FUNCTION_BLOCK MIS_Ctrl
VAR_INPUT
	wNode : WORD; //CANopen nodeID for motor
	ADSNetID : STRING(23); //ADS adress of CANopen master module
	lrUnitConversion : LREAL := 1.0; //Default conversion is 1
END_VAR
VAR_OUTPUT
	stMisMotori : stMisMotor; //Instance of the Mis motor structure
END_VAR
VAR
	bLastEnableMotor : BOOL;//Used to trigger motor enable state 
	iState: INT; //Current state of test
END_VAR

StateHandler(); //handle CANeopen FSA state 
stMisMotori.lrActualUnitPos := ANY_TO_LREAL(stMisMotori.diActualpos) / stMisMotori.lrUnitConversion;//Convert motorcount to units  


CASE iState OF
0:
	stMisMotori.wNodeId := wNode;
	stMisMotori.ADSNetID := ADSNetID;
	stMisMotori.lrUnitConversion := lrUnitConversion; 

END_CASE

METHOD GetState : eDSP402States
VAR_INPUT
END_VAR
//Find the state from the control word
IF (stMisMotori.uiStatus AND 16#4F) = 16#00 THEN
	stMisMotori.State := eDSP402States.NOT_READY_TO_SWITCH_ON;
END_IF;
IF (stMisMotori.uiStatus AND 16#4F) = 16#40 THEN
	stMisMotori.State := eDSP402States.SWITCH_ON_DISABLED;
END_IF;
IF (stMisMotori.uiStatus AND 16#6F) = 16#21 THEN
	stMisMotori.State := eDSP402States.READY_TO_SWITCH_ON;
END_IF;
IF (stMisMotori.uiStatus AND 16#6F) = 16#23 THEN
	stMisMotori.State := eDSP402States.SWITCHED_ON;
END_IF;
IF (stMisMotori.uiStatus AND 16#6F) = 16#27 THEN
	stMisMotori.State := eDSP402States.OPERATION_ENABLE;
END_IF;
IF (stMisMotori.uiStatus AND 16#4F) = 16#0F THEN
	stMisMotori.State:= eDSP402States.FAULT;
END_IF;
IF (stMisMotori.uiStatus AND 16#6F) = 16#07 THEN
	stMisMotori.State := eDSP402States.QUICK_STOP_ACTIVE;
END_IF;
GetState := stMisMotori.State;
END_METHOD

METHOD StateHandler : eDSP402States
VAR_INPUT
END_VAR

VAR
END_VAR


CASE GetState() OF
	
	eDSP402States.NOT_READY_TO_SWITCH_ON:		
	//Should automatically change state
	eDSP402States.SWITCH_ON_DISABLED:
		IF stMisMotori.bEnableMotor THEN 
			stMisMotori.uiCtrWord := 16#06;
		END_IF

	eDSP402States.READY_TO_SWITCH_ON:
		IF stMisMotori.bEnableMotor THEN 
			stMisMotori.uiCtrWord := 16#07;
		ELSE
			stMisMotori.uiCtrWord := 16#06;
		END_IF
			
	eDSP402States.SWITCHED_ON:
		IF stMisMotori.bEnableMotor THEN 
			stMisMotori.uiCtrWord := 16#0F;
		ELSE
			stMisMotori.uiCtrWord := 16#06;
		END_IF
	
	eDSP402States.OPERATION_ENABLE:
		IF stMisMotori.bQuickStop THEN
			stMisMotori.uiCtrWord := 16#02; 
		ELSIF NOT stMisMotori.bEnableMotor THEN 
			stMisMotori.uiCtrWord := 16#06;
		END_IF
	eDSP402States.FAULT:
		IF NOT stMisMotori.bEnableMotor THEN
			stMisMotori.uiCtrWord := ANY_TO_UINT(CSETBIT32(inVal32 := stMisMotori.uiCtrWord,bitNo := 7,bitVal := FALSE)); //Clear reset error
		ELSIF NOT bLastEnableMotor THEN
			stMisMotori.uiCtrWord := ANY_TO_UINT(CSETBIT32(inVal32 := stMisMotori.uiCtrWord,bitNo := 7,bitVal := TRUE)); //reset error
		END_IF
	eDSP402States.QUICK_STOP_ACTIVE:
		IF NOT stMisMotori.bQuickStop THEN
			stMisMotori.uiCtrWord := 16#00;
		END_IF

END_CASE;	
bLastEnableMotor := stMisMotori.bEnableMotor;
END_METHOD

END_FUNCTION_BLOCK
